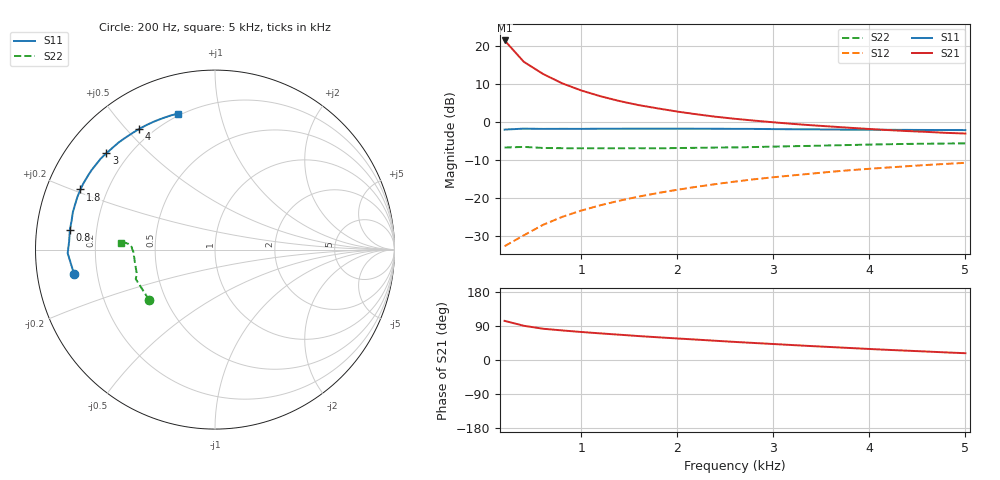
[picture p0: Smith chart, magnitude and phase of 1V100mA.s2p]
#  HZ  S  MA  R  50.0000
! Device:MCH4020
! Bias:VCE=1V, IC=100mA
!MHZ	S11(MAG/ANG)		S21(MAG/ANG)		S12(MAG/ANG)		S22(MAG/ANG)
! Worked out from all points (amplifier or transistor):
!   25 points, 200 Hz to 5 kHz, reference 50 ohm
!   highest |S21| = 21.6 dB at 200 Hz (marker M1)
!   |S21| within 3 dB of that: start of sweep to 306.4 Hz
!   unconditionally stable (mu >= 1): 526.2 Hz to end of sweep
!   at 1 kHz: K = 1.12, MAG = 13.7 dB, |S12| = -23.3 dB
!   at 2.6 kHz: K = 1.12, MAG = 6.1 dB, |S12| = -15.7 dB
!   at 5 kHz: K = 1.08, MAG = 2.1 dB, |S12| = -10.8 dB
!   S11 on the Smith chart (normalised r, x): 200 Hz: 0.11, -0.08; 800 Hz: 0.10, +0.07; 1.8 kHz: 0.10, +0.21; 3 kHz: 0.12, +0.37; 4 kHz: 0.15, +0.54; 5 kHz: 0.19, +0.75
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200  0.797 -170.2  11.99 103.3  0.023 46.0  0.462 -142.7
400  0.821 -178.6  6.267 90.3  0.032 55.8  0.471 -159.7
600  0.814 176.9  4.334 82.5  0.044 60.5  0.456 -162.5
800  0.816 172.4  3.254 78.0  0.056 63.5  0.453 -167.1
1000  0.815 168.6  2.616 73.9  0.068 65.0  0.452 -169.7
1200  0.819 165.2  2.196 70.2  0.08 65.6  0.452 -172.2
1400  0.819 162.0  1.895 66.7  0.092 65.4  0.452 -173.8
1600  0.821 158.9  1.674 63.1  0.104 64.8  0.453 -175.5
1800  0.821 155.9  1.516 59.9  0.116 64.3  0.451 -177.0
2000  0.821 153.3  1.378 56.8  0.128 63.4  0.455 -178.3
2200  0.819 150.2  1.27 53.8  0.14 62.4  0.458 -179.4
2400  0.818 147.4  1.178 50.7  0.152 61.1  0.462 179.5
2600  0.815 144.6  1.107 47.7  0.164 59.7  0.464 178.3
2800  0.814 141.6  1.048 44.9  0.176 58.3  0.469 177.7
3000  0.809 138.5  0.995 42.2  0.187 56.9  0.475 176.9
3200  0.805 135.5  0.949 39.4  0.198 55.3  0.481 176.5
3400  0.803 132.2  0.909 36.7  0.209 53.8  0.486 176.1
3800  0.796 125.6  0.842 31.6  0.232 50.5  0.499 175.7
4000  0.794 122.1  0.812 29.1  0.242 48.7  0.505 175.6
4200  0.792 118.7  0.785 26.7  0.252 47.0  0.511 175.6
4600  0.788 111.8  0.743 22.3  0.272 43.4  0.519 175.8
5000  0.785 105.1  0.707 17.9  0.29 39.9  0.525 175.8
